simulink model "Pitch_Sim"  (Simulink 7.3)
settings: Solver=ode45  StartTime=0.0  StopTime=100  RelTol=1e-3
undefined symbols (not defined in the file or in its folder): Ap, Bp, Cp, Dp, Kq

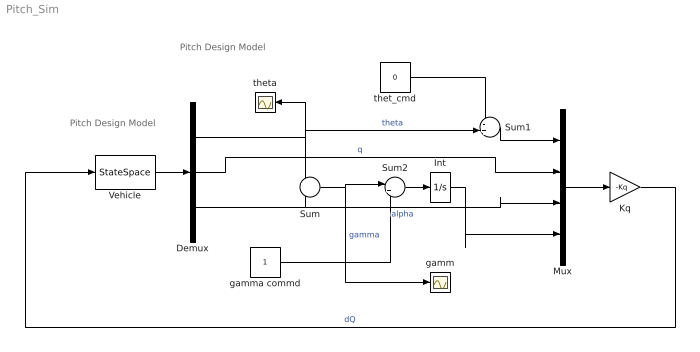
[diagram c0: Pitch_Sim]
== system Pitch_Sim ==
  note: Pitch Design Model
  note: Pitch Design Model
  Demux : Demux  Outputs=3
  Int : Integrator
  Kq : Gain  Gain=-Kq  Multiplication=Matrix(K*u) (u vector)  ParameterDataType=fixdt(1, 16)  ParameterScaling=2^0  OutDataType=fixdt(1, 16)  OutScaling=2^0
  Mux : Mux
  Sum : Sum  Inputs=+-  OutDataType=sfix(16)  OutScaling=2^0
  Sum1 : Sum  Inputs=-+|  OutDataType=sfix(16)  OutScaling=2^0
  Sum2 : Sum  Inputs=|+-  OutDataType=sfix(16)  OutScaling=2^0
  Vehicle : StateSpace  A=Ap  B=Bp  C=Cp  D=Dp
  gamm : Scope
  gamma commd : Constant  OutDataType=fixdt(1, 16)  OutScaling=2^0
  thet_cmd : Constant  Value=0  OutDataType=fixdt(1, 16)  OutScaling=2^0
  theta : Scope
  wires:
  Vehicle/1 -> Demux/1
  Demux/1 -> Sum/1, Sum1/2, theta/1  "theta"
  Demux/2 -> Mux/2  "q"
  Demux/3 -> Sum/2, Mux/3  "alpha"
  Kq/1 -> Vehicle/1  "dQ"
  Sum1/1 -> Mux/1
  thet_cmd/1 -> Sum1/1
  Int/1 -> Mux/4
  Sum/1 -> Sum2/1, gamm/1  "gamma"
  Sum2/1 -> Int/1
  gamma commd/1 -> Sum2/2
  Mux/1 -> Kq/1
